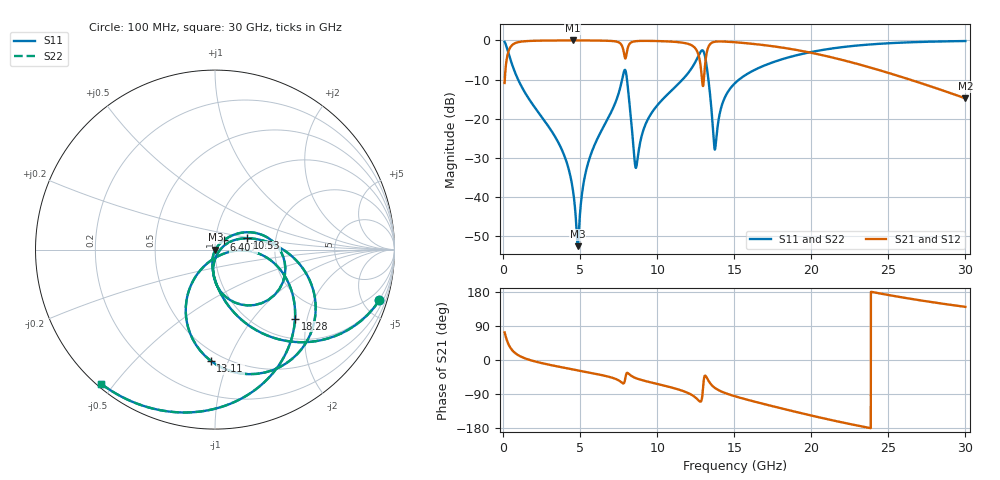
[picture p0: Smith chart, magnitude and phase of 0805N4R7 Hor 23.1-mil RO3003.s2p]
# GHz S MA R 50
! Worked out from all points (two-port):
!   3201 points, 100 MHz to 30 GHz, reference 50 ohm
!   highest |S21| = -0.02 dB at 4.51 GHz (marker M1); lowest = -14.8 dB at 30 GHz (marker M2)
!   |S21| within 3 dB of the highest: 333.5 MHz to 7.834 GHz (7.5 GHz wide, 184 % of centre); 13.22 GHz to 19.81 GHz (6.588 GHz wide, 39.9 % of centre)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
!   lowest |S11| = -52.5 dB at 4.847 GHz (marker M3), VSWR 1.00, Z = 50.2 - j0.111 ohm
!   |S11| at or under -10 dB: 976 MHz to 7.724 GHz (6.748 GHz wide, 155 % of centre); 8.041 GHz to 11.65 GHz (3.604 GHz wide, 36.6 % of centre); 13.32 GHz to 15.31 GHz (1.99 GHz wide, 13.9 % of centre)
!   |S22| runs from -52.5 to -0.2 dB; largest |S21 - S12| = 0
!   S11 on the Smith chart (normalised r, x): 100 MHz: 0.94, -6.49; 6.407 GHz: 1.10, +0.12; 10.53 GHz: 1.43, +0.19; 13.11 GHz: 0.43, -0.87; 18.28 GHz: 1.44, -1.69; 30 GHz: 0.01, -0.46
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0.1  0.9582 -17.2  0.2859 72.8  0.2859 72.8  0.9582 -17.2
0.5298125  0.5313 -60.9  0.8466 29.1  0.8466 29.1  0.5313 -60.9
1.025031  0.3017 -78.1  0.9525 11.7  0.9525 11.7  0.3017 -78.1
3.669313  0.04626 -105.8  0.9969 -18.1  0.9969 -18.1  0.04626 -105.8
4.51025  0.01315 -105.0  0.9975 -24.7  0.9975 -24.7  0.01315 -105.0
4.846625  0.00237 -27.8  0.9975 -27.3  0.9975 -27.3  0.00237 -27.8
5.089563  0.00982 46.0  0.9973 -29.1  0.9973 -29.1  0.00982 46.0
6.407031  0.07197 46.6  0.9928 -39.9  0.9928 -39.9  0.07197 46.6
7.575  0.2384 23.2  0.9257 -55.6  0.9257 -55.6  0.2384 23.2
7.902031  0.4208 -28.5  0.604 -54.3  0.604 -54.3  0.4208 -28.5
8.649531  0.02448 -19.3  0.9782 -48.4  0.9782 -48.4  0.02448 -19.3
10.06978  0.1534 23.2  0.9797 -63.8  0.9797 -63.8  0.1534 23.2
10.52763  0.1917 19.2  0.9729 -68.4  0.9729 -68.4  0.1917 19.2
12.06934  0.3967 -1.7  0.8946 -88.3  0.8946 -88.3  0.3967 -1.7
12.68603  0.6393 -28.7  0.6468 -106.7  0.6468 -106.7  0.6393 -28.7
13.1065  0.6206 -92.1  0.4845 -41.2  0.4845 -41.2  0.6206 -92.1
13.75122  0.04066 -57.3  0.9605 -73.8  0.9605 -73.8  0.04066 -57.3
15.05  0.2847 -8.2  0.9461 -95.8  0.9461 -95.8  0.2847 -8.2
18.28294  0.5885 -40.7  0.7991 -129.9  0.7991 -129.9  0.5885 -40.7
20.03956  0.7132 -57.6  0.6914 -146.9  0.6914 -146.9  0.7132 -57.6
25.01978  0.9189 -99.2  0.3839 171.4  0.3839 171.4  0.9189 -99.2
30  0.9806 -130.3  0.1822 140.2  0.1822 140.2  0.9806 -130.3
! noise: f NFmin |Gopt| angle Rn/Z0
0.1  0.0007567  0.9196  1.258  0.002079
3.417  0.005944  0.6887  19.55  0.003609
6.743  0.01518  0.7555  37.37  0.01128
10.06  0.0212  0.748  54.58  0.01344
13.39  0.09033  0.9165  71.44  0.1575
16.7  0.0297  0.7256  85.25  0.01189
20.03  0.03565  0.7366  98.5  0.01189
23.35  0.04658  0.773  111.4  0.01377
26.67  0.06409  0.8194  124.2  0.01684
30  0.09369  0.8687  137.1  0.02117
